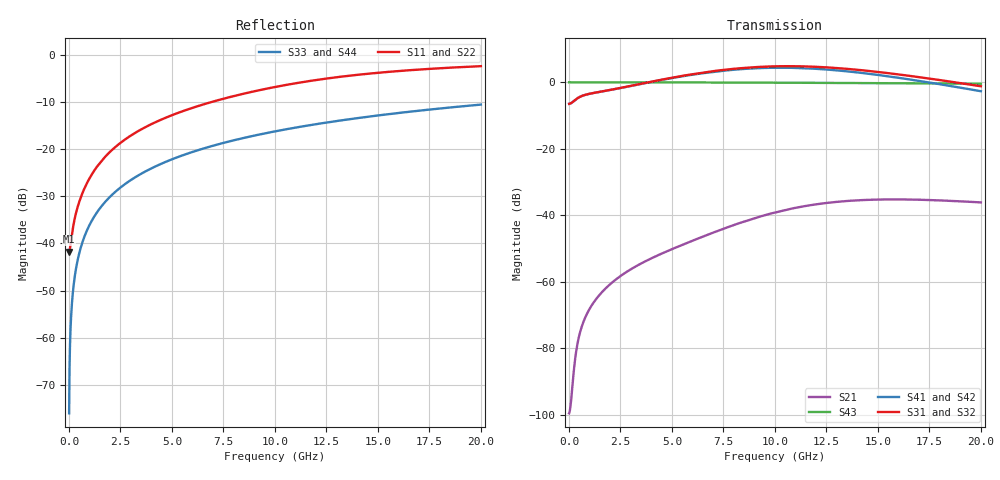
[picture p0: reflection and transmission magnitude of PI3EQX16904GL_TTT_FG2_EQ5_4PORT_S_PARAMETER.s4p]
! NPort=4 DATA=2000 NOISE=0 GROUPDELAY=0 COMPLEX_DATAFORMAT=POLAR
! NumOfBlock=1 NumOfParam=0
! .MODEL Smodel S TSTONEFILE=PI3EQX16904GL_TTT_FG2_EQ5_4PORT_S_PARAMETER.s4p TYPE=S
!  -- The above .MODEL line can be used for the S element in the netlist.
! The s parameter is extracted from the linear redriver, it is not bi-directional; only s(4,1)s(4,2) and s(3,1)s(3,2)
! should be the insertion loss
!Port definition:
!Port1 = input+
!Port2 = input-
!Port3 = output+
!Port4 = output-
# Hz S MA R  50
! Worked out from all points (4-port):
!   2000 points, 10 MHz to 20 GHz, reference 50 ohm
!   strongest paths, dB at 10 MHz, 5.01 GHz, 10.01 GHz, 15.01 GHz, 20 GHz:
!     S31: -6.5, 1.4, 4.8, 3.1, -1.2
!     S32: -6.5, 1.2, 4.6, 3.0, -1.3
!     S41: -6.5, 1.3, 4.4, 2.2, -2.7
!     S42: -6.5, 1.1, 4.2, 2.1, -2.8
!     S43: 0.0, 0.0, -0.1, -0.3, -0.4
!     S21: -99.6, -50.2, -39.1, -35.3, -36.1
!   lowest |S11| = -41.7 dB at 10 MHz (marker M1), VSWR 1.02, Z = 49.2 - j0.0603 ohm
!   |S11| at or under -10 dB: start of sweep to 6.888 GHz
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1e7  0.008182 -175.7  1.05e-05 7.7  0 0.0  0 0.0
     1.05e-05 7.7  0.008182 -175.7  0 0.0  0 0.0
     0.4743 0.5  0.4743 -179.5  0.0001571 -90.0  1 -0.0
     0.4743 -179.6  0.4743 0.4  1 -0.0  0.0001571 -90.0
3.9e8  0.02299 -119.3  0.0001056 117.8  0 0.0  0 0.0
       0.0001056 117.8  0.02299 -119.3  0 0.0  0 0.0
       0.5695 10.3  0.5692 -169.8  0.006126 -90.4  1 -0.4
       0.5695 -170.4  0.5692 9.5  1 -0.4  0.006126 -90.4
1.63e9  0.07746 -102.7  0.0007112 107.3  0 0.0  0 0.0
        0.000711 107.3  0.07746 -102.7  0 0.0  0 0.0
        0.7315 3.5  0.73 -176.9  0.02559 -91.5  0.9996 -1.5
        0.7305 -179.4  0.729 0.2  0.9996 -1.5  0.02559 -91.5
6.07e9  0.2788 -105.0  0.004257 94.1  0 0.0  0 0.0
        0.004224 94.3  0.2787 -105.1  0 0.0  0 0.0
        1.336 -38.3  1.308 141.2  0.09488 -95.7  0.9951 -5.4
        1.312 130.9  1.284 -49.6  0.9951 -5.4  0.09488 -95.7
9.85e9  0.452 -112.4  0.0108 65.9  0 0.0  0 0.0
        0.01071 66.7  0.4517 -112.4  0 0.0  0 0.0
        1.734 -98.3  1.701 81.7  0.1528 -99.1  0.9873 -8.8
        1.654 64.6  1.623 -115.5  0.9873 -8.8  0.1528 -99.1
1.389e10  0.6145 -122.7  0.01678 19.0  0 0.0  0 0.0
          0.01669 20.2  0.6141 -122.7  0 0.0  0 0.0
          1.554 -166.2  1.529 13.7  0.2128 -102.8  0.9752 -12.3
          1.42 -9.7  1.397 170.2  0.9752 -12.3  0.2128 -102.8
2e10  0.7641 -136.1  0.01564 -35.5  0 0.0  0 0.0
      0.01561 -33.8  0.764 -136.1  0 0.0  0 0.0
      0.8718 108.3  0.8579 -71.9  0.2986 -108.1  0.9506 -17.4
      0.7341 -103.6  0.7224 76.2  0.9506 -17.4  0.2986 -108.1
